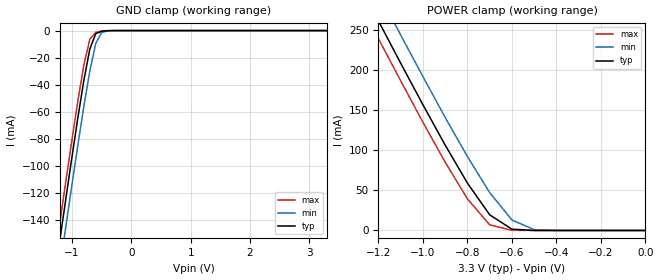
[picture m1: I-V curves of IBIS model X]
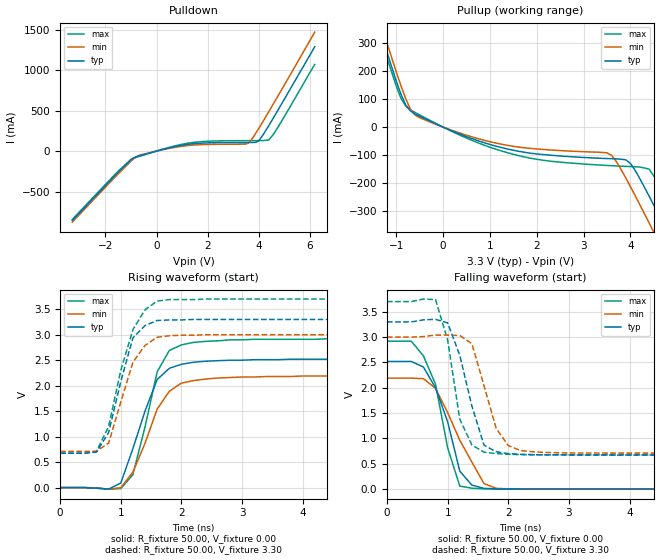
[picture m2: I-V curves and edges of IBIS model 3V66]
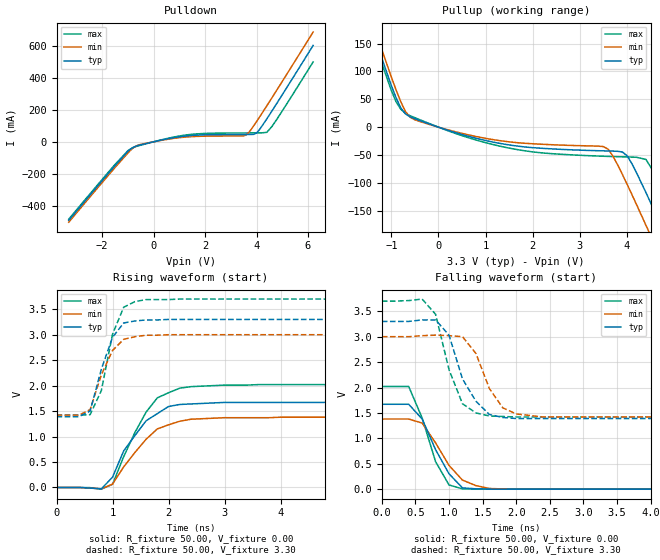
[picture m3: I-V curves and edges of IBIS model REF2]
|   * 9250-12.ibs * IBIS 2.1 Model for ICS9250-12
| Rev History
| Rev No.   Description
| 1.0   Initial release with Updated Parasitic Parameters
[IBIS Ver]   2.1
[Comment char]  |_char
[File name]   9250-12.ibs
[Date]   Aug 15, 2002
[File Rev]   1.1
[Source]   Originated at Integrated Circuit Systems, Inc.
[Disclaimer]
(C) Copyright Integrated Circuit Systems, Inc. 1997
   All rights reserved
ICS hereby grants the user of this IBIS model a non-exclusive,
nontransferable license to use this IBIS model under the following terms.
Before using this IBIS model, the user should read this license.
If the user does not accept these terms,  the IBIS model should be
returned to ICS within 30 days.
   The user is granted this license only to use the IBIS model and
is not granted rights to sell, load, rent, lease or license the IBIS
model in whole or in part, or in modified form to anyone other than
user. User may modify the IBIS model to suit its specific
applications but rights to derivative works and such modifications
shall belong to ICS.
   This IBIS model is provided on an "AS IS" basis and ICS makes
absolutely no warranty with respect to the information contained
herein. ICS DISCLAIMS AND CUSTOMER WAIVES ALL WARRANTIES, EXPRESS
OR IMPLIED, INCLUDING WARRANTIES OF MERCHANTABILITY OR FITNESS FOR
A PARTICULAR PURPOSE. The entire risk as to quality and performance
is with the Customer. ACCORDINGLY, IN NO EVENT SHALL THE COMPANY BE
LIABLE FOR ANY DAMAGES, WHETHER IN CONTRACT OR TORT,INCLUDING ANY
LOST PROFITS OR OTHER INCIDENTAL, CONSEQUENTIAL, EXEMPLARY, OR
PUNITIVE DAMAGES ARISING OUT OF THE USE OR APPLICATION OF THE IBIS
model provided in this package. Further, ICS reserves the right to
make changes without notice to any product herein to improve
reliability, function, or design. ICS does not convey any license
under patent rights or any other intellectual property rights,
including those of third parties.
   ICS is not obligated to provide maintenance or support
for the licensed IBIS model.
|   COMPONENT: ICS9250-12
[Component]   ICS9250-12
[Manufacturer]  ICS
[Package]
| variable   typ   min   max
R_pkg   81.1m   62.2m   100.0m
L_pkg   6.7nH   4.9nH   8.5nH
C_pkg   0.53pF  0.21pF  0.85pF
[Pin]   signal_name   model_name   R_pin   L_pin   C_pin
1   GNDREF   GND
2   REF0   REF2
3   REF1   REF2
4   VDDREF   POWER
5   X1   X
6   X2   X
7   GNDPCI   GND
8   PCICLK_F   PCICLK
9   PCICLK1   PCICLK
10   VDDPCI   POWER
11   PCICLK2   PCICLK
12   PCICLK3   PCICLK
13   GNDPCI   GND
14   PCICLK4   PCICLK
15   PCICLK5   PCICLK
16   VDDPCI   POWER
17   PCICLK6   PCICLK
18   PCICLK7   PCICLK
19   GNDPCI   GND
20   GND66   GND
21   3V66_0   3V66
22   3V66_1   3V66
23   VDD66   POWER
24   GND66   GND
25   3V66_2   3V66
26   3V66_3   3V66
27   VDD66   POWER
28   SEL133/100#   SEL133/100
29   GND48   GND
30   48MHz   48MHz3
31   VDD48   POWER
32   SEL0   SEL
33   SEL1   SEL
34   SPREAD#   SPREAD
35   PD#   PD
36   CPU_STOP#   CPUSTOP
37   PCI_STOP#   PCISTOP
38   GNDCOR   GND
39   VDDCOR   POWER
40   GNDLCPU   GND
41   CPUCLK0   CPU1
42   CPUCLK1   CPU1
43   VDDLCPU   POWER
44   GNDLCPU   GND
45   CPUCLK2   CPU1
46   CPUCLK3   CPU1
47   VDDLCPU   POWER
48   GNDLCPU/2   GND
49   CPU/2_0   CPU1
50   CPU/2_1   CPU1
51   VDDLCPU   POWER
52   GNDLIOAPIC   GND
53   IOAPIC0   IOAPIC1
54   IOAPIC1   IOAPIC1
55   IOAPIC2   IOAPIC1
56   VDDLIOAPIC   POWER
| Models and submodels in the file (13): X (Input), 3V66 (Output), REF2 (Output), 48MHz3 (Output), PCICLK (Output), CPUSTOP (Input), PCISTOP (Input), SEL (Input), PD (Input), SEL133/100 (Input), SPREAD (Input), CPU1 (Output), IOAPIC1 (Output)
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|*  Either 3.3V or 2.5V
|** All model are simulated with typical corner process
|   Model X
[Model]   X
Model_type   Input
Polarity   Non-Inverting
Vinl = 800.00mV
Vinh =   2.00V
C_comp   5.50pF   5.00pF   6.00pF
[Temperature Range]   27.00   70.00   0.00
[Voltage Range]   3.30V   3.00V   3.70V
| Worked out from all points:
|   GND clamp passes 1 mA (typ) near -0.53 V on its own axis
|   POWER clamp passes 1 mA (typ) near -0.56 V on its own axis
[GND_clamp]
| voltage   I(typ)   I(min)   I(max)
-3.3V     -818.7mA   -838.4mA   -806.5mA
-1.3V     -184.4mA   -205.1mA   -171.6mA
-1.2V     -153.6mA   -174.3mA   -140.8mA
-1.1V     -123.2mA   -143.8mA   -110.3mA
-1V       -93.23mA   -113.8mA   -80.48mA
-900mV    -64.14mA   -84.35mA   -51.7mA
-800mV    -36.72mA   -56.02mA   -25.33mA
-700mV    -13.63mA   -29.93mA   -6.41mA
-600mV    -2.31mA    -9.53mA    -1.31mA
-500mV    -487.9uA   -1.36mA    -326.3uA
-400mV    -91uA      -228.6uA   -44.4uA
3.3V      108.9pA    1.5uA      48.42pA
[POWER_clamp]
| voltage   I(typ)   I(min)   I(max)
-3.3V     1.41A      1.44A      1.39A
-1.3V     314.3mA    349.5mA    292.4mA
-1.2V     261.1mA    296.3mA    239.1mA
-1.1V     208.4mA    243.6mA    186.5mA
-1V       156.6mA    191.7mA    134.8mA
-900mV    106.3mA    140.8mA    85.01mA
-800mV    58.94mA    92.02mA    39.34mA
-700mV    19.46mA    47.14mA    7mA
-600mV    1.61mA     13.03mA    241.9uA
-500mV    48.08uA    1.03mA     4.48uA
-400mV    1.09uA     42.41uA    71.42nA
0V        108.9pA    1.22nA     66.46pA
|   Model 3V66
[Model]   3V66
Model_type   Output
Polarity   Non-Inverting
Vmeas = 1.5V
Cref = 30pF
Rref = 0
Vref = 1.5V
C_comp   5.50pF   5.00pF   6.00pF
[Temperature Range]   27.00   70.00   0.00
[Voltage Range]   3.30V   3.00V   3.70V
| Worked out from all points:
|   slope of the pulldown table from 0 to 0.495 V, typ, clamps not added: 12.4 ohm
|   slope of the pullup table from 0 to 0.495 V, typ, clamps not added: 14.7 ohm
|   rising waveform, R_fixture 50.00, V_fixture 0.00: 20-80 % time 444ps typ, 474ps min, 361ps max; typ from 0 V to 2.52 V
|   rising waveform, R_fixture 50.00, V_fixture 3.30: 20-80 % time 338ps typ, 377ps min, 384ps max; typ from 0.674 V to 3.3 V
|   falling waveform, R_fixture 50.00, V_fixture 0.00: 20-80 % time 377ps typ, 546ps min, 357ps max; typ from 2.52 V to 0 V
|   falling waveform, R_fixture 50.00, V_fixture 3.30: 20-80 % time 356ps typ, 339ps min, 278ps max; typ from 3.3 V to 0.674 V
[Pulldown]
| voltage   I(typ)   I(min)   I(max)
-3.3V     -857.9mA   -878.4mA   -845.3mA
-1.5V     -261.3mA   -282.1mA   -248.7mA
-1V       -107.9mA   -125mA     -102.2mA
-700mV    -61.18mA   -54.61mA   -68.48mA
400mV     32.81mA    27.49mA    37.39mA
1.3V      86.08mA    70.47mA    101mA
3.6V      106.5mA    98.57mA    128.8mA
3.9V      108.8mA    225.9mA    129.5mA
4V        126.6mA    276.5mA    129.7mA
4.4V      314.9mA    487.2mA    137.4mA
4.8V      527.7mA    703mA      316.3mA
6.2V      1.29A      1.47A      1.07A
[Pullup]
| voltage   I(typ)   I(min)   I(max)
-3.3V     1.4A       1.43A      1.38A
-1.5V     421.2mA    455.2mA    400.3mA
-900mV    116.5mA    146.2mA    102mA
-700mV    57.52mA    63.85mA    61.81mA
-500mV    38.48mA    33.44mA    43.28mA
1.4V      -78.79mA   -65.56mA   -92.19mA
3.5V      -111.7mA   -91.56mA   -136.3mA
4V        -128.7mA   -211.2mA   -140.2mA
4.4V      -245.1mA   -340.5mA   -149.2mA
4.8V      -375.8mA   -472.8mA   -260.1mA
5.2V      -509mA     -606.4mA   -391.1mA
6.2V      -845.7mA   -943.1mA   -726.8mA
[Ramp]
| variable   typ   min   max
dV/dt_r   1.51/354.04p   1.31/416.22p   1.75/312.34p
dV/dt_f   1.58/300.00p   1.37/300.00p   1.81/300.00p
[Rising Waveform]
R_fixture = 50.00
V_fixture = 0.00
V_fixture_min = 0.00
V_fixture_max = 0.00
| time   V(typ)   V(min)   V(max)
0s        0V         0V         0V
800ps     -31.01mV   -29.88mV   -31.17mV
1ns       89.14mV    -3.03mV    -19.9mV
1.2ns     765.6mV    303mV      254mV
1.4ns     1.5V       870.1mV    1.19V
1.6ns     2.12V      1.54V      2.27V
1.8ns     2.34V      1.89V      2.69V
2ns       2.42V      2.05V      2.8V
3.4ns     2.51V      2.18V      2.91V
10ns      2.52V      2.19V      2.92V
[Rising Waveform]
R_fixture = 50.00
V_fixture = 3.30
V_fixture_min = 3.00
V_fixture_max = 3.70
| time   V(typ)   V(min)   V(max)
0s        673.6mV    711.3mV    675.9mV
400ps     673.6mV    711.3mV    675.9mV
600ps     696.8mV    712.9mV    712.6mV
800ps     1.08V      874mV      1.2V
1ns       2.08V      1.68V      2.3V
1.2ns     2.94V      2.46V      3.1V
1.4ns     3.18V      2.79V      3.49V
1.6ns     3.28V      2.95V      3.66V
2.4ns     3.3V       3V         3.7V
10ns      3.3V       3V         3.7V
[Falling Waveform]
R_fixture = 50.00
V_fixture = 0.00
V_fixture_min = 0.00
V_fixture_max = 0.00
| time   V(typ)   V(min)   V(max)
0s        2.52V      2.19V      2.92V
400ps     2.52V      2.19V      2.92V
600ps     2.41V      2.18V      2.63V
800ps     2V         1.99V      2.07V
1ns       1.33V      1.51V      817.2mV
1.2ns     355.4mV    965.6mV    60.84mV
1.4ns     79.4mV     534.8mV    19.11mV
1.6ns     15.91mV    109mV      7.22mV
1.8ns     6.17mV     16.27mV    3.69mV
10ns      0V         1.56uV     652.7nV
[Falling Waveform]
R_fixture = 50.00
V_fixture = 3.30
V_fixture_min = 3.00
V_fixture_max = 3.70
| time   V(typ)   V(min)   V(max)
0s        3.3V       3V         3.7V
800ps     3.35V      3.04V      3.74V
1ns       3.28V      3.04V      2.94V
1.2ns     2.64V      3.03V      1.38V
1.4ns     1.64V      2.87V      871.5mV
1.6ns     866.9mV    2.04V      731.3mV
1.8ns     737.7mV    1.2V       700.7mV
2ns       701.1mV    861.1mV    687.7mV
2.2ns     687.2mV    761.6mV    681.9mV
10ns      673.6mV    711.3mV    675.9mV
|   Model REF2
[Model]   REF2
Model_type   Output
Polarity   Non-Inverting
Vmeas = 1.5V
Cref = 20pF
Rref = 0
Vref = 1.5V
C_comp   5.50pF   5.00pF   6.00pF
[Temperature Range]   27.00   70.00   0.00
[Voltage Range]   3.30V   3.00V   3.70V
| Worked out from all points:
|   slope of the pulldown table from 0 to 0.495 V, typ, clamps not added: 28.9 ohm
|   slope of the pullup table from 0 to 0.495 V, typ, clamps not added: 37.7 ohm
|   rising waveform, R_fixture 50.00, V_fixture 0.00: 20-80 % time 586ps typ, 631ps min, 572ps max; typ from 0 V to 1.67 V
|   rising waveform, R_fixture 50.00, V_fixture 3.30: 20-80 % time 323ps typ, 337ps min, 299ps max; typ from 1.39 V to 3.3 V
|   falling waveform, R_fixture 50.00, V_fixture 0.00: 20-80 % time 372ps typ, 432ps min, 329ps max; typ from 1.67 V to 0 V
|   falling waveform, R_fixture 50.00, V_fixture 3.30: 20-80 % time 355ps typ, 337ps min, 306ps max; typ from 3.3 V to 1.39 V
[Pulldown]
| voltage   I(typ)   I(min)   I(max)
-3.3V     -490.2mA   -501.8mA   -482.9mA
-1.5V     -148.6mA   -160.5mA   -141.3mA
-1V       -59.86mA   -70.16mA   -55.59mA
-700mV    -28.18mA   -27.69mA   -30.26mA
300mV     10.71mA    9mA        12.18mA
1.3V      36.89mA    30.2mA     43.26mA
3.6V      45.65mA    42.52mA    55.18mA
3.9V      46.6mA     102mA      55.47mA
4V        54.75mA    125.7mA    55.57mA
4.4V      142.8mA    224.3mA    59.01mA
4.8V      242.4mA    325.4mA    142.6mA
6.2V      601mA      684.6mA    498.1mA
[Pullup]
| voltage   I(typ)   I(min)   I(max)
-3.3V     655.7mA    671.1mA    646.1mA
-1.5V     196.6mA    212.6mA    186.7mA
-900mV    53.14mA    67.41mA    45.92mA
-600mV    18.38mA    17.65mA    20.45mA
1.4V      -30.61mA   -25.38mA   -35.92mA
3.5V      -42.6mA    -34.96mA   -52.28mA
3.7V      -43.04mA   -51.97mA   -52.84mA
4V        -51.32mA   -102.4mA   -53.55mA
4.4V      -117.3mA   -176.1mA   -57.95mA
4.8V      -191.7mA   -251.5mA   -120.6mA
5.2V      -267.5mA   -327.7mA   -195mA
6.2V      -459.4mA   -519.6mA   -386.1mA
[Ramp]
| variable   typ   min   max
dV/dt_r   1.00/537.02p   825.60m/558.03p   1.21/485.76p
dV/dt_f   1.15/300.00p   947.40m/300.00p   1.37/300.00p
[Rising Waveform]
R_fixture = 50.00
V_fixture = 0.00
V_fixture_min = 0.00
V_fixture_max = 0.00
| time   V(typ)   V(min)   V(max)
0s        0V         0V         0V
800ps     -28.09mV   -26.46mV   -33.51mV
1ns       201.9mV    65.4mV     62.89mV
1.2ns     719.4mV    405.4mV    606.7mV
1.6ns     1.31V      947.4mV    1.48V
1.8ns     1.45V      1.15V      1.76V
2ns       1.59V      1.23V      1.86V
2.2ns     1.63V      1.3V       1.95V
3ns       1.67V      1.37V      2.01V
10ns      1.67V      1.38V      2.02V
[Rising Waveform]
R_fixture = 50.00
V_fixture = 3.30
V_fixture_min = 3.00
V_fixture_max = 3.70
| time   V(typ)   V(min)   V(max)
0s        1.39V      1.42V      1.42V
400ps     1.39V      1.42V      1.42V
600ps     1.5V       1.53V      1.43V
800ps     2.32V      2.21V      1.9V
1ns       2.95V      2.69V      3.01V
1.2ns     3.23V      2.91V      3.54V
1.4ns     3.27V      2.96V      3.65V
1.6ns     3.29V      2.99V      3.69V
2.2ns     3.3V       3V         3.7V
10ns      3.3V       3V         3.7V
[Falling Waveform]
R_fixture = 50.00
V_fixture = 0.00
V_fixture_min = 0.00
V_fixture_max = 0.00
| time   V(typ)   V(min)   V(max)
0s        1.67V      1.38V      2.02V
400ps     1.67V      1.38V      2.02V
600ps     1.38V      1.3V       1.4V
800ps     776.5mV    909.8mV    540.5mV
1ns       301.6mV    467mV      82.21mV
1.2ns     24.9mV     177.7mV    5.7mV
1.4ns     7.06mV     69.84mV    596.7uV
1.6ns     1.53mV     13.67mV    397.9uV
1.8ns     -199.7uV   3.91mV     131uV
10ns      2.28uV     6.21uV     0V
[Falling Waveform]
R_fixture = 50.00
V_fixture = 3.30
V_fixture_min = 3.00
V_fixture_max = 3.70
| time   V(typ)   V(min)   V(max)
0s        3.3V       3V         3.7V
600ps     3.33V      3.02V      3.74V
800ps     3.33V      3.03V      3.44V
1ns       3.03V      3.02V      2.35V
1.2ns     2.17V      3V         1.68V
1.4ns     1.73V      2.67V      1.5V
1.6ns     1.47V      1.98V      1.44V
1.8ns     1.41V      1.6V       1.43V
2.4ns     1.39V      1.42V      1.42V
10ns      1.39V      1.42V      1.42V
